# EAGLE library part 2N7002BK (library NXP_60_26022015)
60 V, 340 mA dual N-channel Trench MOSFET Dual N-channel enhancement mode Field-Effect Transistor (FET) in an ultra small SOT666 Surface-Mounted Device (SMD) plastic package using Trench MOSFET technology. AAL Eindhoven MK
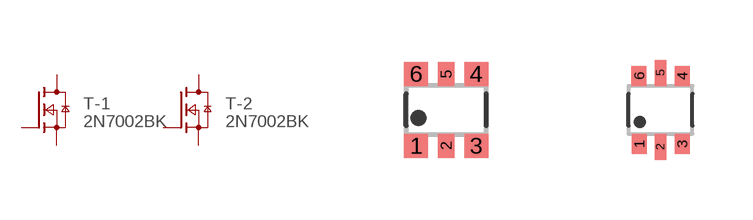
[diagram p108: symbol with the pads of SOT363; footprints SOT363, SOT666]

Designator prefix T; gates -1=N-MOSFET -2=N-MOSFET

## 2N7002BKS  [SOT363]
1  -1:S  pas
2  -1:G  pas
3  -2:D  pas
4  -2:S  pas
5  -2:G  pas
6  -1:D  pas

## 2N7002BKV  [SOT666]
Pads as for SOT363

## Footprint SOT363 (pad centres in mm)
SOT363 Plastic surface-mounted package; 6 leads JEDEC: -- IEC: -- JEITA: SC-88
smd 0.6 x 0.6: 1 -0.75,-0.9; 3 0.75,-0.9; 4 0.75,0.9; 6 -0.75,0.9
smd 0.4 x 0.6: 2 0,-0.9; 5 0,0.9

## Footprint SOT666 (pad centres in mm)
SOT 666 Reflow soldering foorprint Source: Philips - BAS70_1PS7XSB70_SER_8.pdf
smd 0.375 x 0.5: 1 -0.537,-0.85; 3 0.538,-0.85; 4 0.538,0.85; 6 -0.538,0.85
smd 0.3 x 0.65: 2 0,-0.925; 5 0,0.925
